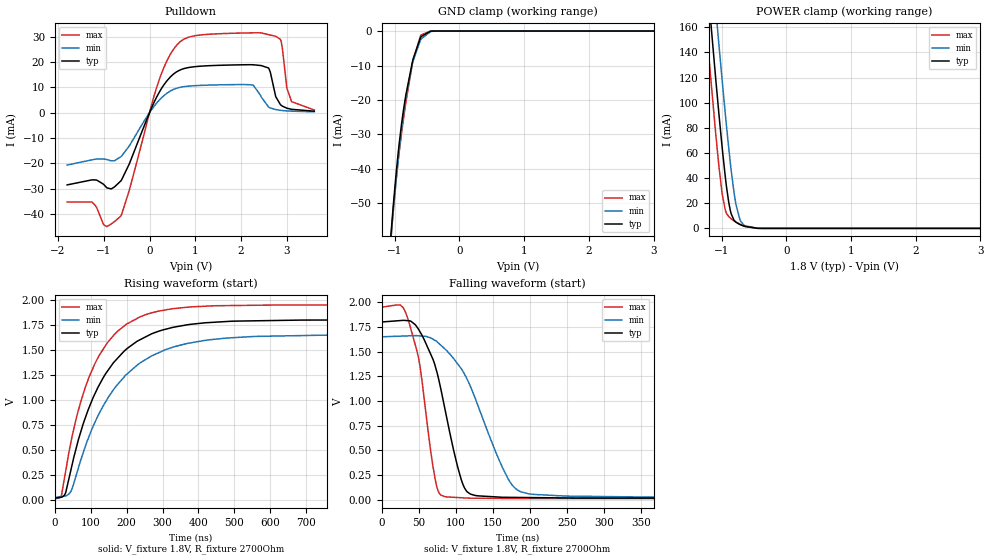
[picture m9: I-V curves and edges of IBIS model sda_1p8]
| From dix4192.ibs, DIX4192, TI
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|   sda_1p8 Model
[Model]   sda_1p8
Model_type   I/O_open_drain
Polarity   Non-Inverting
Enable   Active-Low
Vinl = 0.54
Vinh = 1.26
Vmeas = 0.9
Vref = 1.8
Cref = 2pF
Rref = 2000
|   typ   min   max
C_comp   31.7425pF   25.9201pF   37.6391pF
|C_comp_pulldown   31.7419pF   25.9193pF   37.6391pF
[Model spec]
|subparameter
Vinl   0.54   0.495   0.585
Vinh   1.26   1.155   1.365
| Where nom  PVT is Nominal Process, 1.8V, 27C
|   Fast PVT is Strong Process,  1.95V, -40C
|   Slow PVT is Weak Process,   1.65V, 105C
[Voltage Range]   1.8   1.65   1.95
[Temperature Range]   27   105   -40
[Pullup Reference]   1.8   1.65   1.95
[Pulldown Reference]   0   -0   -0
[Power Clamp Reference]   1.8   1.65   1.95
[GND Clamp Reference]   0   0   0
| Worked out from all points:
|   slope of the pulldown table from 0 to 0.27 V, typ, clamps not added: 27.6 ohm
|   GND clamp passes 1 mA (typ) near -0.53 V on its own axis
|   POWER clamp passes 1 mA (typ) near -0.56 V on its own axis
|   falling waveform, V_fixture 1.8V, R_fixture 2700Ohm: 20-80 % time 33.3ns typ, 54.1ns min, 22.5ns max; typ from 1.8 V to 0.015 V
|   rising waveform, V_fixture 1.8V, R_fixture 2700Ohm: 20-80 % time 132ns typ, 154ns min, 109ns max; typ from 0.015 V to 1.8 V
[Pulldown]
|   Voltage   I(typ)   I(min)   I(max)
-1.8V     -28.48mA   -20.66mA   -35.2mA
-1.26V    -26.5mA    -18.6mA    -35.21mA
-936mV    -29.56mA   -18.48mA   -44.92mA
-628.2mV  -26.95mA   -17.41mA   -40.76mA
262.8mV   9.565mA    5.875mA    15.49mA
840.6mV   17.76mA    10.46mA    29.68mA
2.266V    18.89mA    10.87mA    31.49mA
2.601V    17.62mA    2.222mA    30.77mA
2.758V    6.313mA    1.228mA    30.13mA
2.882V    2.839mA    891.3uA    27.64mA
3.103V    1.326mA    592.4uA    4.358mA
3.6V      583.4uA    334uA      1.045mA
[GND Clamp]
|   Voltage   I(typ)   I(min)   I(max)
-1.8V     -269.5mA   -244.4mA   -304.6mA
-1.076V   -63.64mA   -64.2mA    -65.25mA
-1.028V   -52.24mA   -53.82mA   -53.43mA
-979.2mV  -41.88mA   -44.02mA   -43.51mA
-930.6mV  -32.88mA   -35mA      -35.28mA
-892.8mV  -26.95mA   -28.67mA   -29.64mA
-828mV    -18.71mA   -19.53mA   -20.92mA
-714.6mV  -8.146mA   -8.682mA   -8.428mA
-590.4mV  -1.599mA   -2.281mA   -1.13mA
-444.6mV  -52.32uA   -160.2uA   -14.34uA
-358.2mV  -3.674uA   -21.45uA   -306.9nA
3.6V      0A         0A         0A
[POWER Clamp]
|   Voltage   I(typ)   I(min)   I(max)
-1.8V     564.8mA    620.9mA    520.8mA
-1.233V   204.8mA    261.9mA    159.6mA
-1.168V   165.5mA    222.3mA    120.5mA
-1.087V   117.7mA    173.8mA    74.13mA
-1.039V   90.27mA    145.4mA    48.83mA
-984.6mV  61.6mA     114.7mA    25.82mA
-941.4mV  40.98mA    91.12mA    14.65mA
-887.4mV  20.49mA    63.43mA    9.326mA
-806.4mV  6.463mA    28.45mA    6.043mA
-714.6mV  3.048mA    6.727mA    3.292mA
-412.2mV  29.86uA    75.19uA    8.803uA
3.6V      0A         0A         0A
[Ramp]
R_load = 2700
|   typ   min   max
dV/dt_r   1.07092/1.31103e-07   0.976558/1.53189e-07   1.16389/1.09057e-07
dV/dt_f   1.07092/3.3104e-08   0.976558/5.40894e-08   1.16389/2.23478e-08
[Falling Waveform]
V_fixture = 1.8V
V_fixture_min = 1.65V
V_fixture_max = 1.95V
R_fixture = 2700Ohm
C_fixture = 0F
|   Time   V(typ)   V(min)   V(max)
0s        1.8V       1.65V      1.95V
34.34ns   1.814V     1.659V     1.856V
51.31ns   1.706V     1.659V     1.372V
72.69ns   1.343V     1.611V     189.9mV
85ns      934mV      1.529V     31.82mV
102.5ns   333.7mV    1.377V     21.97mV
115.6ns   78.51mV    1.216V     16.4mV
171ns     23.87mV    207.9mV    12.38mV
198.1ns   21.76mV    60.43mV    11.21mV
1.25us    15.13mV    22.37mV    10.19mV
[Rising Waveform]
V_fixture = 1.8V
V_fixture_min = 1.65V
V_fixture_max = 1.95V
R_fixture = 2700Ohm
C_fixture = 0F
|   Time   V(typ)   V(min)   V(max)
0s        15.13mV    22.37mV    10.19mV
18.56ns   25.46mV    31.97mV    44.85mV
30.72ns   74.6mV     38.73mV    293.7mV
44.14ns   285.5mV    78.67mV    561.3mV
72.69ns   683.1mV    401.8mV    985.7mV
111.7ns   1.06V      774mV      1.362V
167.3ns   1.387V     1.12V      1.659V
238.5ns   1.603V     1.371V     1.832V
478.6ns   1.784V     1.618V     1.943V
1.25us    1.8V       1.65V      1.95V
